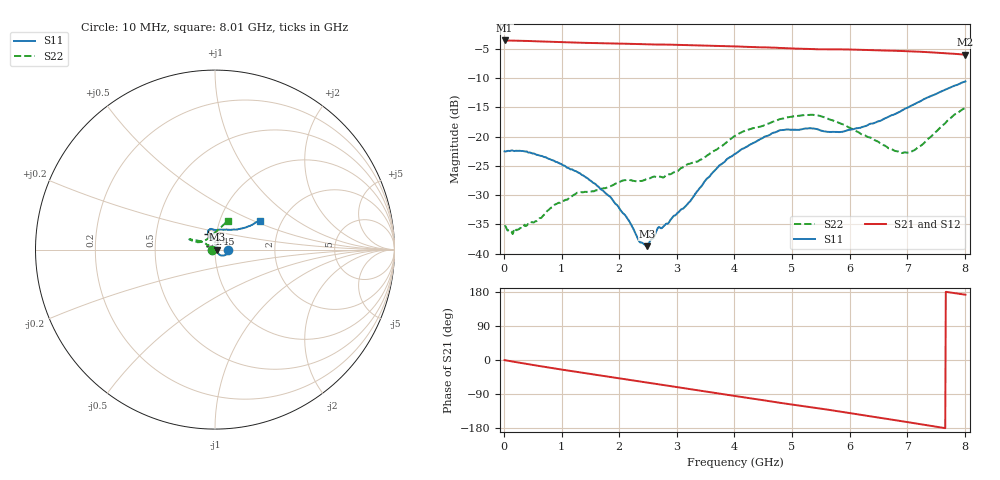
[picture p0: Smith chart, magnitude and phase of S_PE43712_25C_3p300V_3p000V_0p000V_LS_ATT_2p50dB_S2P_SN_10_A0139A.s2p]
! DEVICE ID: PE43712
! File Path: z:\PE43713\PE43713_CHAR_NOM_04292014\AMB\3p300\LS_ATT_2p50dB\PE43713_AMB_3p300V_3p000V_0p000V_LS_ATT_2p50dB_S2P_SN_10_A0139A.s2p
! Serial: 10
! Lot: A0139A
! Temp: 25C
! VDD: 3.300
! VSS: 0.000
! Control_Hi: 3.000
! Control_Lo: 0.000
! Attenuation Step: 2.50dB
! Port 1: RF1
! Port 2: RF2
! ThroughPath:1-2
! IDD: 0.0001468006
! ISS: -7.97e-008
#  Hz  S  RI  R  50
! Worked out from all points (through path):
!   801 points, 10 MHz to 8.01 GHz, reference 50 ohm
!   highest |S21| = -3.54 dB at 10 MHz (marker M1); lowest = -6.0 dB at 8.01 GHz (marker M2)
!   group delay of S21, straight-line fit = 64.3 ps
!   lowest |S11| = -38.7 dB at 2.48 GHz (marker M3), VSWR 1.02, Z = 51.2 - j0.0477 ohm
!   |S11| at or under -10 dB: start of sweep to end of sweep
!   |S22| runs from -36.7 to -15.1 dB; largest |S21 - S12| = 0.0019
!   S11 on the Smith chart (normalised r, x): 10 MHz: 1.16, -0.00; 4.45 GHz: 0.91, +0.16; 8.01 GHz: 1.54, +0.55
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1e7  0.0748 -0.000431  0.6653 -0.00388  0.665 -0.00362  -0.0171 -8.83e-05
1.2e8  0.0758 -0.00499  0.6628 -0.0378  0.6626 -0.0378  -0.0156 -0.0007
2.8e8  0.074 -0.0152  0.6554 -0.0859  0.655 -0.0861  -0.0156 -0.00541
7e8  0.0607 -0.0282  0.6192 -0.2011  0.6189 -0.2009  -0.0193 -0.00952
9.1e8  0.0516 -0.032  0.594 -0.2533  0.594 -0.2531  -0.0238 -0.0118
1.35e9  0.0338 -0.0328  0.5309 -0.3496  0.5308 -0.3495  -0.0316 -0.0112
1.85e9  0.0199 -0.0229  0.4444 -0.4424  0.4444 -0.4422  -0.0376 -0.00243
2.14e9  0.0129 -0.0153  0.387 -0.4881  0.3871 -0.4878  -0.0426 0.00348
2.35e9  0.0112 -0.00591  0.3422 -0.5166  0.3423 -0.5165  -0.0407 0.00947
2.48e9  0.0115 -0.000467  0.3134 -0.5317  0.3134 -0.5317  -0.0404 0.0159
2.68e9  0.0129 0.0106  0.2695 -0.5513  0.2697 -0.5513  -0.0369 0.0268
3.14e9  0.00223 0.025  0.1601 -0.5869  0.1602 -0.5868  -0.0471 0.0297
3.39e9  -0.00238 0.0358  0.0993 -0.5952  0.0993 -0.5953  -0.0528 0.0339
3.72e9  -0.00968 0.0546  0.0197 -0.5972  0.0196 -0.5971  -0.0679 0.0413
4.01e9  -0.0211 0.068  -0.0511 -0.59  -0.0508 -0.5899  -0.0892 0.0485
4.45e9  -0.0382 0.0874  -0.1497 -0.5619  -0.1498 -0.5625  -0.1111 0.0508
4.8e9  -0.0364 0.1077  -0.225 -0.5284  -0.2245 -0.5286  -0.1305 0.0551
5.35e9  -0.0221 0.1155  -0.3239 -0.4589  -0.3238 -0.4585  -0.143 0.0573
5.86e9  0.0115 0.109  -0.4061 -0.3829  -0.4052 -0.383  -0.119 0.0483
6.68e9  0.0986 0.1109  -0.4973 -0.2212  -0.497 -0.221  -0.0644 0.0464
7.1e9  0.1454 0.117  -0.521 -0.1276  -0.5205 -0.1276  -0.0272 0.0706
8.01e9  0.2489 0.1618  -0.4986 0.0678  -0.4971 0.0669  0.0698 0.1618
